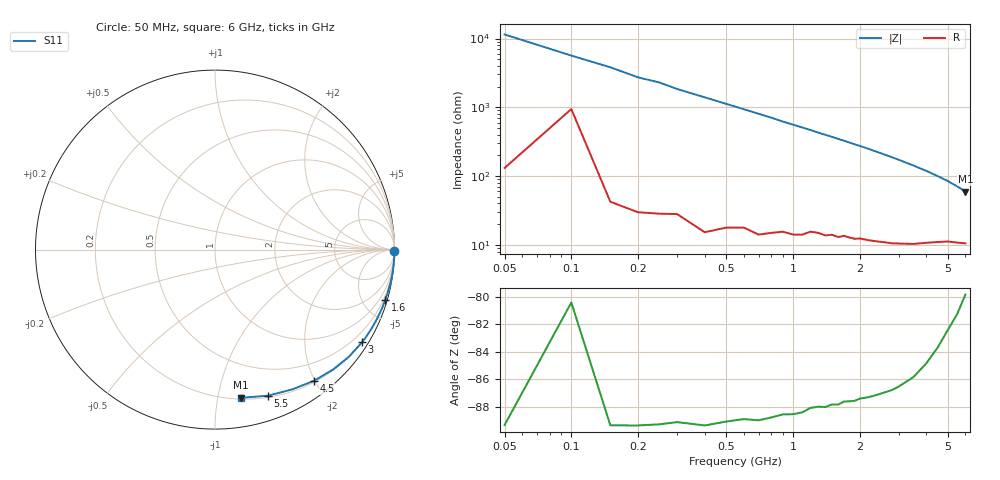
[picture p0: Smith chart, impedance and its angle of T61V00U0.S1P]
! SIEMENS Discrete & RF Semiconductors
! BAT62
! Si Schottky Diode in SOT143
! VR = 1 V
! S-Parameters:  February  1997
# GHz  S  MA  R  50
!  f  S11
! GHz  MAG  ANG
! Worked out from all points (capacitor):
!   34 points, 50 MHz to 6 GHz, reference 50 ohm
!   read as one part to ground: C = 278 fF near 50 MHz
!   lowest |Z| = 59.4 ohm at 6 GHz (marker M1)
!   S11 on the Smith chart (normalised r, x): 50 MHz: open; 1.6 GHz: 0.26, -6.93; 3 GHz: 0.21, -3.45; 4.5 GHz: 0.22, -1.99; 5.5 GHz: 0.22, -1.41; 6 GHz: 0.21, -1.17
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0.05  0.9999 -0.5
0.1  0.997 -1.0
0.15  0.9997 -1.5
0.2  0.9996 -2.1
0.25  0.9995 -2.5
0.3  0.9992 -3.1
0.4  0.9992 -4.1
0.7  0.9978 -7.1
0.8  0.997 -8.1
0.9  0.996 -9.2
1.1  0.9947 -11.2
1.4  0.9915 -14.3
1.5  0.9901 -15.3
1.6  0.9895 -16.4
1.7  0.9877 -17.4
1.9  0.9859 -19.6
2  0.9843 -20.6
2.2  0.9819 -22.8
2.4  0.979 -25.1
2.6  0.9758 -27.4
2.8  0.9725 -29.8
3  0.9683 -32.2
3.5  0.9555 -38.7
4  0.9375 -45.5
4.5  0.9155 -53.0
5  0.89 -61.0
5.5  0.866 -70.0
6  0.8386 -80.0
